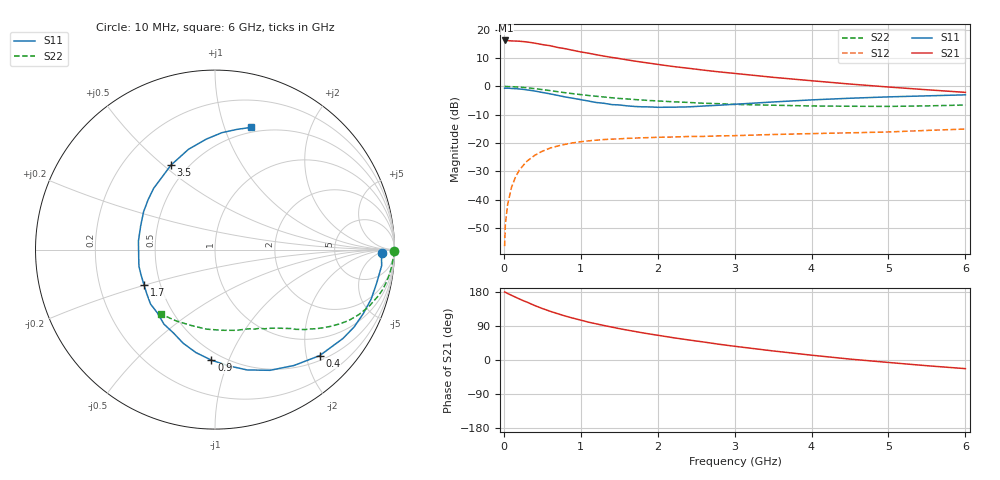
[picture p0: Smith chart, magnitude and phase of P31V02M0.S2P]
! SIEMENS Small Signal Semiconductors
! BFP181
! Si NPN RF Bipolar Junction Transistor in SOT143
! VCE = 1 V  IC = 2 mA
! Common Emitter S-Parameters:  March  1996
# GHz  S  MA  R  50
!  f  S11  S21  S12  S22
! GHz  MAG  ANG  MAG  ANG  MAG  ANG  MAG  ANG
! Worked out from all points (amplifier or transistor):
!   36 points, 10 MHz to 6 GHz, reference 50 ohm
!   highest |S21| = 16.2 dB at 20 MHz (marker M1)
!   |S21| within 3 dB of that: start of sweep to 813.6 MHz
!   unconditionally stable (mu >= 1): 2.265 GHz to end of sweep
!   at 250 MHz: K = 0.13, MSG = 21.9 dB, |S12| = -28.0 dB
!   at 1.4 GHz: K = 0.69, MSG = 14.4 dB, |S12| = -18.6 dB
!   at 6 GHz: K = 1.21, MAG = 3.7 dB, |S12| = -15.1 dB
!   S11 on the Smith chart (normalised r, x): 10 MHz: 25, -8; 400 MHz: 0.60, -2.26; 900 MHz: 0.44, -0.87; 1.7 GHz: 0.41, -0.20; 3.5 GHz: 0.41, +0.53; 6 GHz: 0.45, +1.23
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0.01  0.9287 -1.3  6.449 179.3  0.0015 89.5  0.996 -0.5
0.02  0.9285 -2.5  6.486 178.7  0.0037 85.8  0.9995 -1.1
0.05  0.9329 -5.5  6.444 175.4  0.0083 88.8  0.9934 -2.8
0.1  0.9197 -11.8  6.361 170.7  0.0165 82.3  0.9891 -5.4
0.15  0.9127 -17.6  6.335 165.9  0.0247 79.1  0.9813 -8.2
0.25  0.8869 -29.1  6.19 156.7  0.0398 72.5  0.9605 -13.4
0.3  0.868 -34.8  6.11 152.8  0.0475 69.4  0.9458 -15.8
0.4  0.8298 -45.4  5.814 143.8  0.0603 63.1  0.9136 -20.4
0.5  0.7815 -55.7  5.486 135.9  0.0715 57.5  0.8787 -24.4
0.6  0.7391 -65.5  5.244 128.7  0.0811 52.5  0.8427 -28.0
0.8  0.6505 -83.7  4.633 115.9  0.0949 44.2  0.7728 -33.6
0.9  0.6161 -91.9  4.337 110.4  0.1006 40.9  0.743 -35.9
1.1  0.5509 -108.8  3.861 99.9  0.1089 35.1  0.6908 -39.8
1.4  0.4771 -132.2  3.259 87.0  0.117 28.5  0.6301 -44.8
1.7  0.4419 -153.5  2.804 75.5  0.1219 24.5  0.5857 -48.6
1.9  0.4338 -167.6  2.564 68.5  0.1246 22.1  0.5624 -51.1
2.2  0.4293 173.7  2.247 58.9  0.1275 19.6  0.5345 -55.1
2.8  0.4649 143.3  1.805 41.5  0.1335 15.9  0.495 -63.6
3.5  0.5306 117.6  1.447 23.9  0.1412 13.1  0.465 -75.3
4.5  0.6175 94.5  1.1 2.4  0.1512 9.1  0.4457 -96.2
5.5  0.6807 79.7  0.872 -15.1  0.1667 7.4  0.4525 -118.7
6  0.709 73.7  0.784 -22.8  0.1764 5.3  0.4687 -130.0
